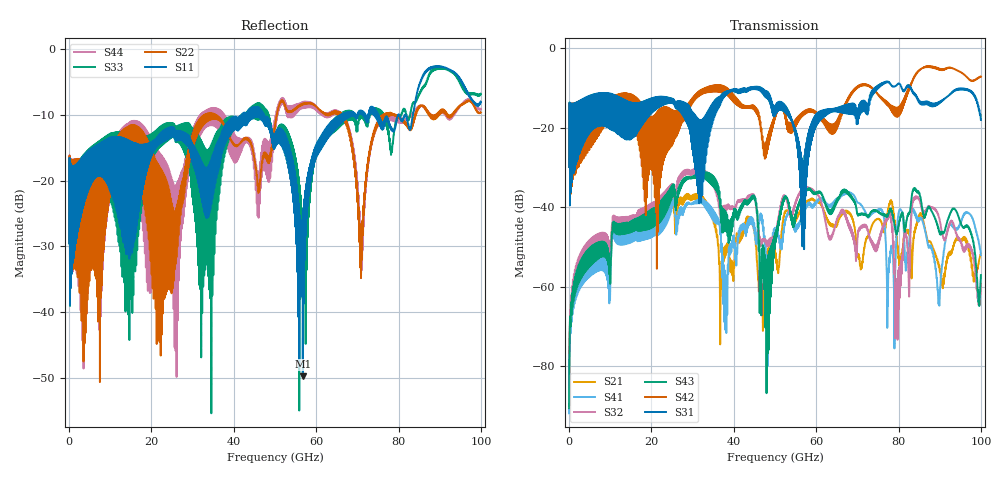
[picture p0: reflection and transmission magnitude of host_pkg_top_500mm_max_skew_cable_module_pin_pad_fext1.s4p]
# Hz S RI R 50
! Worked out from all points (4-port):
!   10000 points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, 10 MHz to 100 GHz, reference 50 ohm
!   strongest paths, dB at 10 MHz, 25.01 GHz, 50.01 GHz, 75.01 GHz, 100 GHz:
!     S31: -29.9, -12.7, -14.7, -9.8, -18.1
!     S42: -29.9, -15.8, -16.8, -11.6, -7.2
!     S43: -90.6, -37.2, -46.7, -41.3, -57.1
!     S32: -88.9, -36.5, -46.6, -50.1, -59.4
!     S41: -91.9, -40.0, -45.6, -40.8, -52.1
!     S21: -89.9, -40.1, -52.2, -43.0, -51.8
!   lowest |S11| = -49.8 dB at 56.76 GHz (marker M1), VSWR 1.01, Z = 50 + j0.325 ohm
!   |S11| at or under -10 dB: start of sweep to 42.03 GHz; 47.29 GHz to 66.07 GHz (18.77 GHz wide, 33.1 % of centre); 75.05 GHz to 79.99 GHz (4.936 GHz wide, 6.37 % of centre)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
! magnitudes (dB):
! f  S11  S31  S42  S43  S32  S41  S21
! 10 MHz  -29.5  -29.9  -29.9  -90.6  -88.9  -91.9  -89.9
! 28 GHz  -14.2  -16.0  -17.9  -32.7  -30.8  -39.8  -37.3
! 37.93 GHz  -13.6  -11.8  -10.3  -41.2  -40.1  -69.5  -51.3
! 46.96 GHz  -10.5  -10.9  -22.2  -54.4  -48.1  -43.1  -61.6
! 56.76 GHz  -49.8  -29.1  -17.0  -37.1  -35.5  -42.1  -39.9
! 70.89 GHz  -9.9  -13.6  -9.5  -41.8  -44.9  -39.4  -55.2
! 100 GHz  -8.1  -18.1  -7.2  -57.1  -59.4  -52.1  -51.8
